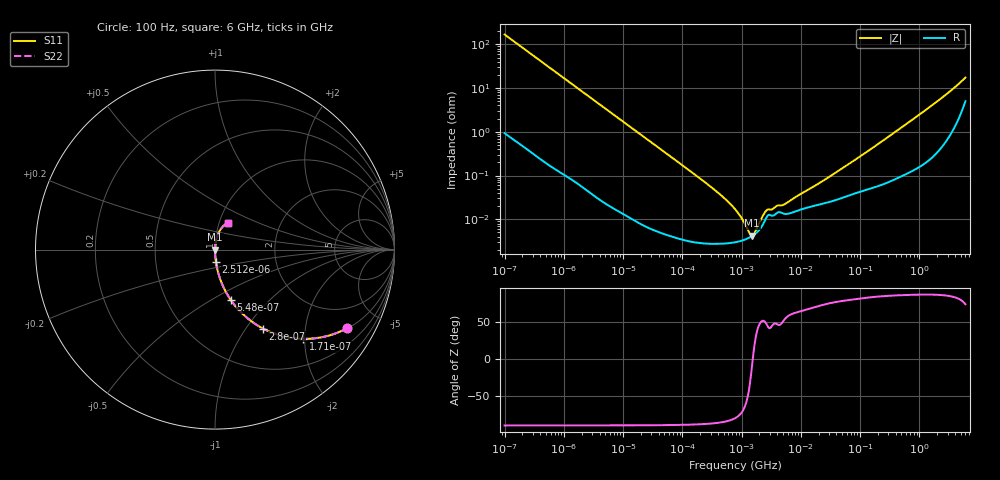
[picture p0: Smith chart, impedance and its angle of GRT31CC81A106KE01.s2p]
!Murata Part Number: GRT31CC81A106KE01
!These Parameters are Measured in Series Mode Connection
!Data Generated on Jun 19, 2026
!  o--ll--o
!Port1  Port2
!  o------o
!Operation Temp=25[degC], DC Bias Voltage=0[V]
!Freq. Start=100[Hz] Stop=6[GHz] 401[Steps]
# Hz S RI R 50
!Freq.(Hz) S11(Real) S11(Imag) S21(Real) S21(Imag) S12(Real) S12(Imag) S22(Real) S22(Imag)
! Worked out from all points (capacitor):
!   401 points, 100 Hz to 6 GHz, reference 50 ohm
!   read as one part in series: C = 9.44 uF near 109 Hz
!   lowest |Z| = 4.19 mohm at 1.516 MHz (marker M1)
!   series resonance near 1.548 MHz, so ESL is about 1.1 nH
!   S11 on the Smith chart (normalised r, x): 100 Hz: 1.02, -3.37; 171 Hz: 1.01, -1.97; 280 Hz: 1.01, -1.21; 548 Hz: 1.00, -0.62; 2.512 kHz: 1.00, -0.14; 6 GHz: 1.10, +0.34
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100  0.738 -0.4369  0.262 0.4369  0.262 0.4369  0.738 -0.4369
171  0.4928 -0.4972  0.5072 0.4972  0.5072 0.4972  0.4928 -0.4972
280  0.2681 -0.4401  0.7319 0.4401  0.7319 0.4401  0.2681 -0.4401
548  0.0885 -0.2811  0.9115 0.2811  0.9115 0.2811  0.0885 -0.2811
1026  0.0276 -0.1607  0.9724 0.1607  0.9724 0.1607  0.0276 -0.1607
2008  0.00768 -0.0841  0.9923 0.0841  0.9923 0.0841  0.00768 -0.0841
2512  0.00502 -0.0675  0.995 0.0675  0.995 0.0675  0.00502 -0.0675
40335  6.87e-05 -0.00427  0.9999 0.00427  0.9999 0.00427  6.87e-05 -0.00427
330837  2.76e-05 -0.0005  1 0.0005  1 0.0005  2.76e-05 -0.0005
541393  2.8e-05 -0.000282  1 0.000282  1 0.000282  2.8e-05 -0.000282
774597  2.97e-05 -0.000168  1 0.000168  1 0.000168  2.97e-05 -0.000168
1059725  3.31e-05 -8.76e-05  1 8.76e-05  1 8.76e-05  3.31e-05 -8.76e-05
1516199  4.16e-05 -4.6e-06  1 4.6e-06  1 4.6e-06  4.16e-05 -4.6e-06
1983483  5.69e-05 5.86e-05  0.9999 -5.86e-05  0.9999 -5.86e-05  5.69e-05 5.86e-05
2713602  0.000117 0.000116  0.9999 -0.000116  0.9999 -0.000116  0.000117 0.000116
5311619  0.000133 0.000176  0.9999 -0.000176  0.9999 -0.000176  0.000133 0.000176
1.555665e7  0.000198 0.000498  0.9998 -0.000498  0.9998 -0.000498  0.000198 0.000498
7.129496e7  0.000369 0.00197  0.9996 -0.00197  0.9996 -0.00197  0.000369 0.00197
3.124326e8  0.000782 0.00794  0.9992 -0.00794  0.9992 -0.00794  0.000782 0.00794
1.873145e9  0.00515 0.0459  0.9948 -0.0459  0.9948 -0.0459  0.00515 0.0459
3.8344e9  0.0211 0.0959  0.9789 -0.0959  0.9789 -0.0959  0.0211 0.0959
6e9  0.0713 0.1482  0.9287 -0.1482  0.9287 -0.1482  0.0713 0.1482
